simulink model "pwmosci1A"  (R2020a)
settings: Solver=VariableStepDiscrete  StartTime=0.0  StopTime=100  MaxStep=1  RelTol=1e-3  EnableMultiTasking=on

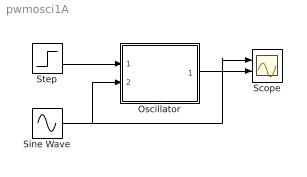
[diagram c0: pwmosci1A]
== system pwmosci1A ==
  Oscillator : Subsystem  mask(PWM-Oszillator){}
      mask help: Oszillator, der ein Rechtecksignal mit variabler Frequenz und Pulsweite erzeugt
  Scope : Scope  NumInputPorts=2
  Sine Wave : Sin  Amplitude=40  Bias=50  Frequency=0.12  Phase=-pi/2  SampleTime=0
  Step : Step  Time=50  Before=0.1  After=0.4  SampleTime=0  ZeroCross=off
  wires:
  Oscillator/1(Out) -> Scope/2
  Sine Wave/1 -> Scope/1, Oscillator/2(In2)
  Step/1 -> Oscillator/1(In1)

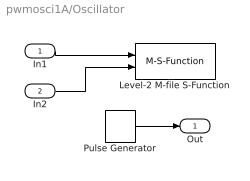
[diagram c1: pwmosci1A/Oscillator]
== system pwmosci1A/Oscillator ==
  In1 : Inport
  In2 : Inport  Port=2
  Level-2 M-file S-Function : M-S-Function  FunctionName=sfun_pwmosciA
  Pulse Generator : DiscretePulseGenerator  PulseType=Time based  Period=2.5  PulseWidth=16.2458
  Out : Outport
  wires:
  In1/1 -> Level-2 M-file S-Function/1
  Pulse Generator/1 -> Out/1
  In2/1 -> Level-2 M-file S-Function/2
